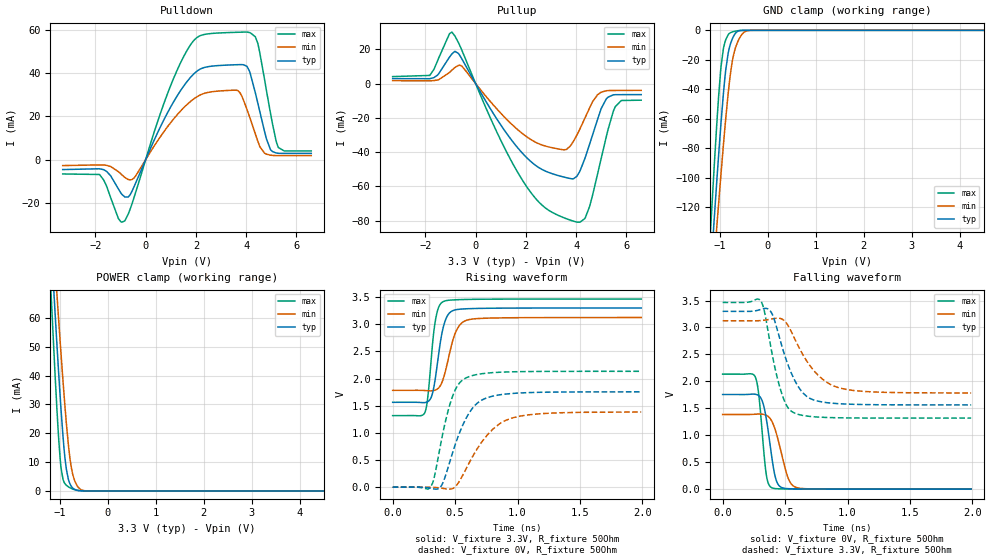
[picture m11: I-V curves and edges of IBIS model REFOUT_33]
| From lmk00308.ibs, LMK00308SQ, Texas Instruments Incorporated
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|   Model REFOUT_33
[Model]   REFOUT_33
Model_type   Output
Polarity   Non-Inverting
Rref =   50.0000
Vref =   1.65
Vmeas =   1.65
|   typ   min   max
C_comp   0.4681pF   0.4606pF   0.4681pF
|Output in low   Nom   Weak   Strong
|C_Comp   0.4681pF   0.4606pF   0.4681pF
|Output in High   Nom   Strong   Weak
|C_Comp High   0.4470pF   0.4470pF   0.4539pF
|Output in Hi-Z   Nom   Strong   Weak
|C_Comp   0.5714pF   0.5375pF   0.5943pF
[Voltage Range]   3.3   3.125   3.465
[Temperature Range]   45   125   -40
[Pullup Reference]   3.3   3.125   3.465
[Pulldown Reference]   0   0   0
[Power Clamp Reference]   3.3   3.125   3.465
[GND Clamp Reference]   0   0   0
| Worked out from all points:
|   slope of the pulldown table from 0 to 0.495 V, typ, clamps not added: 38.4 ohm
|   slope of the pullup table from 0 to 0.495 V, typ, clamps not added: 39.7 ohm
|   GND clamp passes 1 mA (typ) near -0.64 V on its own axis
|   POWER clamp passes 1 mA (typ) near -0.73 V on its own axis
|   falling waveform, V_fixture 0V, R_fixture 50Ohm: 20-80 % time 68.1ps typ, 93.7ps min, 49.6ps max; typ from 1.76 V to 0 V
|   rising waveform, V_fixture 3.3V, R_fixture 50Ohm: 20-80 % time 70.9ps typ, 92.3ps min, 54.2ps max; typ from 1.56 V to 3.3 V
|   rising waveform, V_fixture 0V, R_fixture 50Ohm: 20-80 % time 181ps typ, 249ps min, 131ps max; typ from 0 V to 1.76 V
|   falling waveform, V_fixture 3.3V, R_fixture 50Ohm: 20-80 % time 165ps typ, 231ps min, 121ps max; typ from 3.3 V to 1.56 V
[Pulldown]
|   Voltage   I(typ)   I(min)   I(max)
-3.3V     -4.573mA   -2.732mA   -6.599mA
-1.835V   -4.208mA   -2.432mA   -6.841mA
-825mV    -17.24mA   -8.231mA   -28.18mA
-458.7mV  -12.38mA   -8.451mA   -17.33mA
1.313V    30.49mA    21.48mA    42.8mA
2.64V     43.13mA    31.31mA    58.2mA
3.749V    43.82mA    30.94mA    58.77mA
4.036V    42.97mA    23.03mA    58.82mA
4.363V    30.92mA    11.96mA    56.71mA
4.808V    9.502mA    2.534mA    31.78mA
5.273V    2.937mA    1.849mA    5.759mA
6.59V     2.878mA    1.847mA    3.999mA
[GND Clamp]
|   Voltage   I(typ)   I(min)   I(max)
-3.3V     -1.278A    -1.155A    -1.452A
-1.191V   -165.2mA   -188.8mA   -135.2mA
-1.181V   -160.3mA   -184.5mA   -129.4mA
-1.112V   -126.3mA   -154.6mA   -90.2mA
-1.063V   -102.6mA   -133.7mA   -63.82mA
-973.5mV  -62.6mA    -97.12mA   -24.52mA
-924mV    -42.86mA   -77.76mA   -12.38mA
-874.5mV  -26.59mA   -59.5mA    -6.297mA
-755.7mV  -7.232mA   -24.45mA   -1.307mA
-617.1mV  -551.8uA   -7.168mA   -235.5uA
-409.2mV  -2.249uA   -178.7uA   -1.428uA
6.59V     0A         0A         0A
[Pullup]
|   Voltage   I(typ)   I(min)   I(max)
-3.3V     2.837mA    1.66mA     4.035mA
-1.825V   2.802mA    1.559mA    4.708mA
-943.8mV  17.24mA    7.781mA    29.99mA
-547.8mV  14.38mA    10.1mA     19.41mA
838.2mV   -20.54mA   -14.71mA   -28.09mA
1.957V    -42.12mA   -30.24mA   -58.5mA
3.491V    -54.48mA   -38.65mA   -78.17mA
4.036V    -53.99mA   -29.92mA   -80.86mA
4.531V    -35.62mA   -14.4mA    -71.92mA
4.996V    -14.65mA   -5.088mA   -43.77mA
5.561V    -6.525mA   -4.057mA   -13.49mA
6.59V     -6.465mA   -4.015mA   -9.73mA
[POWER Clamp]
|   Voltage   I(typ)   I(min)   I(max)
-3.3V     764.4mA    683.9mA    872.9mA
-1.181V   85.63mA    98.84mA    67.84mA
-1.102V   62.34mA    78.5mA     41mA
-1.063V   51.11mA    68.55mA    28.62mA
-973.5mV  27.67mA    46.96mA    7.713mA
-914.1mV  14.84mA    33.57mA    3.083mA
-864.6mV  7.506mA    23.45mA    1.948mA
-795.3mV  2.683mA    12.06mA    1.157mA
-726mV    916.9uA    5.383mA    607.1uA
-607.2mV  151.1uA    1.084mA    107.1uA
-438.9mV  3.87uA     23.83uA    2.54uA
6.59V     0A         0A         0A
[Ramp]
R_load = 50
|   typ   min   max
dV/dt_r   1.04193/7.09494e-11   0.804645/9.23387e-11   1.2879/5.41551e-11
dV/dt_f   1.05388/6.8123e-11   0.83142/9.36819e-11   1.28054/4.95818e-11
[Falling Waveform]
V_fixture = 0V
V_fixture_min = 0V
V_fixture_max = 0V
R_fixture = 50Ohm
C_fixture = 0F
|   Time   V(typ)   V(min)   V(max)
0s        1.756V     1.386V     2.134V
260ps     1.762V     1.391V     2.091V
290ps     1.735V     1.394V     1.742V
350ps     1.304V     1.37V      265.7mV
395ps     575.5mV    1.256V     25.11mV
420ps     242.2mV    1.111V     11.58mV
450ps     70.79mV    865.2mV    6.976mV
525ps     9.207mV    203.7mV    3.517mV
590ps     4.717mV    31.53mV    2.2mV
1.99ns    933.1nV    8.119uV    165nV
[Rising Waveform]
V_fixture = 3.3V
V_fixture_min = 3.125V
V_fixture_max = 3.465V
R_fixture = 50Ohm
C_fixture = 0F
|   Time   V(typ)   V(min)   V(max)
0s        1.563V     1.784V     1.319V
260ps     1.56V      1.78V      1.385V
280ps     1.574V     1.776V     1.63V
315ps     1.697V     1.775V     2.529V
340ps     1.981V     1.787V     3.039V
370ps     2.479V     1.833V     3.323V
405ps     2.944V     1.996V     3.418V
500ps     3.265V     2.831V     3.451V
600ps     3.287V     3.08V      3.458V
1.99ns    3.3V       3.125V     3.465V
[Rising Waveform]
V_fixture = 0V
V_fixture_min = 0V
V_fixture_max = 0V
R_fixture = 50Ohm
C_fixture = 0F
|   Time   V(typ)   V(min)   V(max)
0s        5.129nV    9.721nV    4.387nV
305ps     -17.82mV   -737uV     7.758mV
335ps     -33.41mV   -4.285mV   203.6mV
390ps     27.78mV    -17.47mV   857.8mV
470ps     561.9mV    -31.93mV   1.61V
525ps     939.9mV    76.99mV    1.889V
595ps     1.298V     370.4mV    2.021V
760ps     1.651V     967.2mV    2.102V
955ps     1.726V     1.273V     2.125V
1.99ns    1.756V     1.385V     2.134V
[Falling Waveform]
|Gnd
V_fixture = 3.3V
V_fixture_min = 3.125V
V_fixture_max = 3.465V
R_fixture = 50Ohm
C_fixture = 0F
|   Time   V(typ)   V(min)   V(max)
0s        3.3V       3.125V     3.465V
305ps     3.335V     3.129V     3.495V
335ps     3.353V     3.136V     3.296V
390ps     3.278V     3.157V     2.588V
465ps     2.733V     3.166V     1.836V
515ps     2.362V     3.069V     1.543V
575ps     2.03V      2.802V     1.413V
735ps     1.651V     2.187V     1.343V
930ps     1.586V     1.883V     1.325V
1.99ns    1.563V     1.784V     1.319V
